FUNCTION FC 21 : VOID
TITLE =USCITE E COMANDI VARI ASPO/CULLA
VERSION : 0.1

BEGIN
NETWORK
TITLE =INDIETRO ASPO
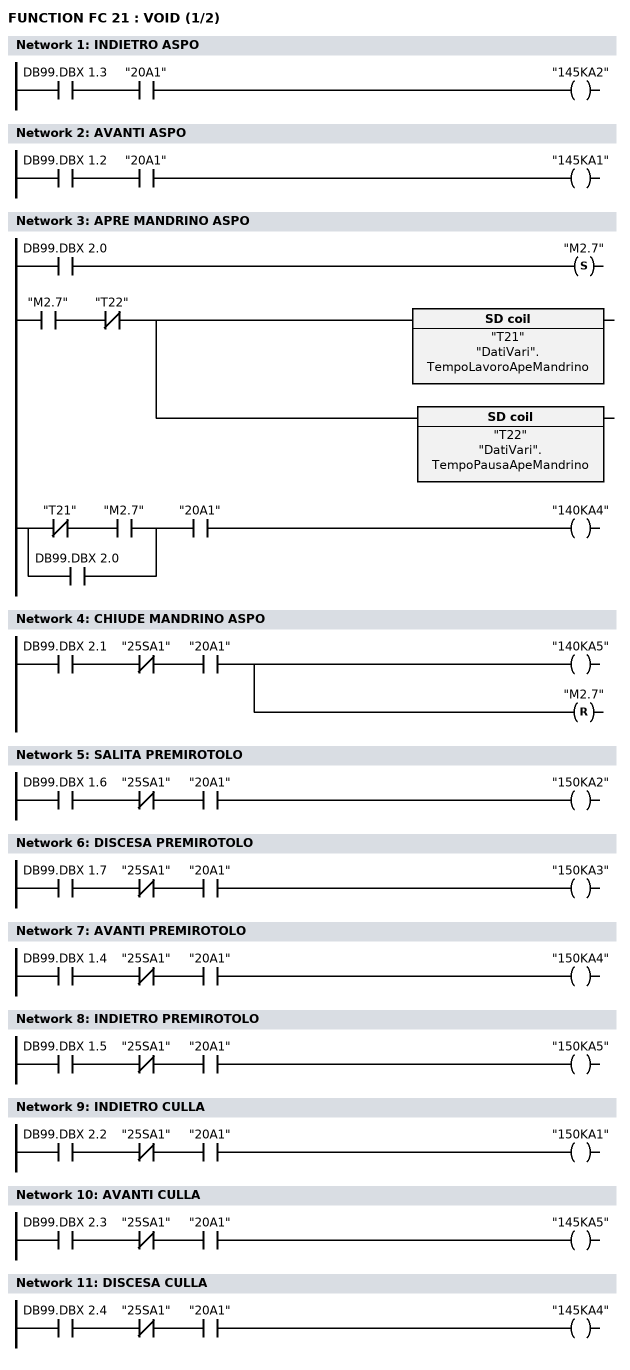
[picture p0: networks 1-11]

      U     DB99.DBX    1.3;
      U     "20A1";
      =     "145KA2";
NETWORK
TITLE =AVANTI ASPO

      U     DB99.DBX    1.2;
      U     "20A1";
      =     "145KA1";
NETWORK
TITLE =APRE MANDRINO ASPO

      U     DB99.DBX    2.0;
      S     "M2.7";

      U     "M2.7";
      UN    "T22";
      L     "DatiVari".TempoLavoroApeMandrino;
      SE    "T21";

      L     "DatiVari".TempoPausaApeMandrino;
      SE    "T22";

      UN    "T21";
      U     "M2.7";
      O     DB99.DBX    2.0;
      U     "20A1";
      =     "140KA4";

NETWORK
TITLE =CHIUDE MANDRINO ASPO

      U     DB99.DBX    2.1;
      UN    "25SA1";
      U     "20A1";
      =     "140KA5";
      R     "M2.7";
NETWORK
TITLE =SALITA PREMIROTOLO

      U     DB99.DBX    1.6;
      UN    "25SA1";
      U     "20A1";
      =     "150KA2";
NETWORK
TITLE =DISCESA PREMIROTOLO

      U     DB99.DBX    1.7;
      UN    "25SA1";
      U     "20A1";
      =     "150KA3";
NETWORK
TITLE =AVANTI PREMIROTOLO

      U     DB99.DBX    1.4;
      UN    "25SA1";
      U     "20A1";
      =     "150KA4";
NETWORK
TITLE =INDIETRO PREMIROTOLO

      U     DB99.DBX    1.5;
      UN    "25SA1";
      U     "20A1";
      =     "150KA5";
NETWORK
TITLE =INDIETRO CULLA

      U     DB99.DBX    2.2;
      UN    "25SA1";
      U     "20A1";
      =     "150KA1";
NETWORK
TITLE =AVANTI CULLA

      U     DB99.DBX    2.3;
      UN    "25SA1";
      U     "20A1";
      =     "145KA5";
NETWORK
TITLE =DISCESA CULLA

      U     DB99.DBX    2.4;
      UN    "25SA1";
      U     "20A1";
      =     "145KA4";
NETWORK
TITLE =SALITA CULLA
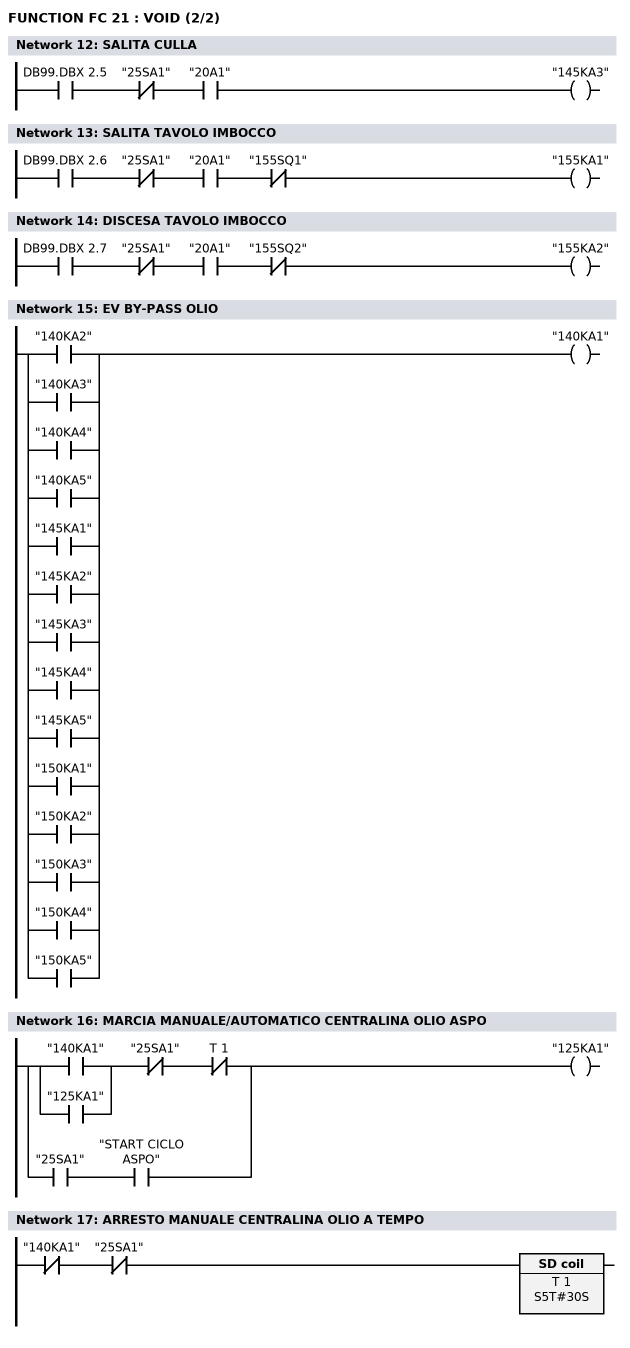
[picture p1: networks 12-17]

      U     DB99.DBX    2.5;
      UN    "25SA1";
      U     "20A1";
      =     "145KA3";
NETWORK
TITLE =SALITA TAVOLO IMBOCCO

      U     DB99.DBX    2.6;
      UN    "25SA1";
      U     "20A1";
      UN    "155SQ1";
      =     "155KA1";
NETWORK
TITLE =DISCESA TAVOLO IMBOCCO

      U     DB99.DBX    2.7;
      UN    "25SA1";
      U     "20A1";
      UN    "155SQ2";
      =     "155KA2";
NETWORK
TITLE =EV BY-PASS OLIO

      O     "140KA2";
      O     "140KA3";
      O     "140KA4";
      O     "140KA5";
      O     "145KA1";
      O     "145KA2";
      O     "145KA3";
      O     "145KA4";
      O     "145KA5";
      O     "150KA1";
      O     "150KA2";
      O     "150KA3";
      O     "150KA4";
      O     "150KA5";
//      O     "155KA1"
//      O     "155KA2"
      =     "140KA1";
NETWORK
TITLE =MARCIA MANUALE/AUTOMATICO CENTRALINA OLIO ASPO

      U(    ;
      O     "140KA1";
      O     "125KA1";
      )     ;
      UN    "25SA1";
      UN    T      1;
      O     ;
      U     "25SA1";
      U     "START CICLO ASPO";
      =     "125KA1";
NETWORK
TITLE =ARRESTO MANUALE CENTRALINA OLIO A TEMPO

      UN    "140KA1";
      UN    "25SA1";
      L     S5T#30S;
      SE    T      1;
NETWORK
TITLE =SEGNALAZIONE ACUSTICA/VISIVA MOVIMENTO CULLA

      UN    "T24";
      L     S5T#1S;
      SE    "T23";

      U     "T23";
      SE    "T24";

      U     "145KA3";
      O     "145KA4";
      O     "145KA5";
      O     "150KA1";
      =     "415KA1";

      U     "415KA1";
      U     "T23";
      =     "A14.0";

END_FUNCTION

